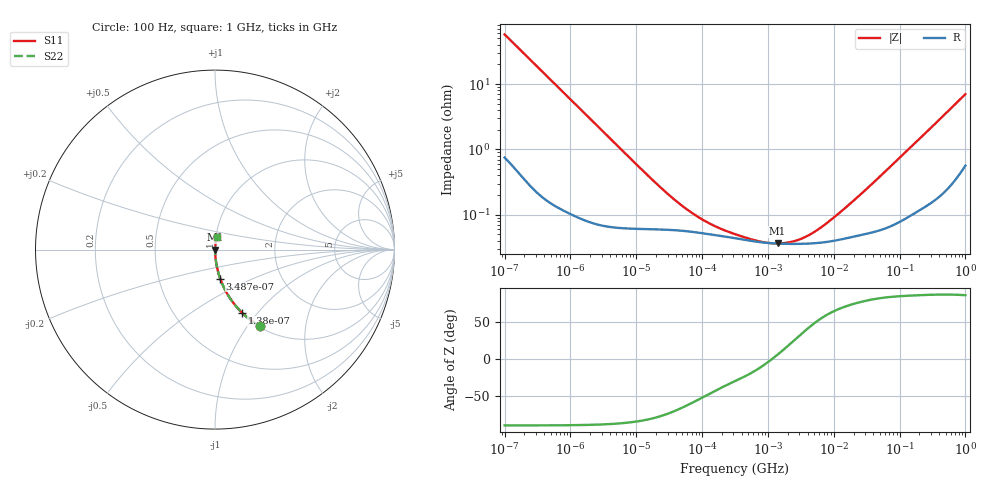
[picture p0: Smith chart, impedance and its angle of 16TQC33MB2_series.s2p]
!  *** S-Parameter ***
!  Copyright (C) Panasonic Industry
!  Conductive Polymer Tantalum Solid Capacitor (POSCAP)
!  Parts No. 16TQC33MB2
!  Connection Mode : Series
!  1  o---||---o  2
!  GND o--------o GND
!  Conditions : Temperature = 20 degC  DC Bias = 0 V
! Frequency Range : 100Hz  -  1GHz  [ 401 Steps ]
# Hz S RI R 50
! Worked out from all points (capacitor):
!   401 points, 100 Hz to 1 GHz, reference 50 ohm
!   read as one part in series: C = 27.6 uF near 108.4 Hz
!   lowest |Z| = 36.3 mohm at 1.404 MHz (marker M1)
!   series resonance near 1.165 MHz, so ESL is about 680 pH
!   S11 on the Smith chart (normalised r, x): 100 Hz: 1.01, -1.15; 138 Hz: 1.01, -0.84; 348.7 Hz: 1.00, -0.33; 1 GHz: 1.01, +0.14
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100  0.2518 -0.4276  0.7482 0.4276  0.7482 0.4276  0.2518 -0.4276
138.0384  0.1522 -0.353  0.8478 0.353  0.8478 0.353  0.1522 -0.353
206.538  0.0756 -0.2585  0.9244 0.2585  0.9244 0.2585  0.0756 -0.2585
348.7386  0.0288 -0.1615  0.9712 0.1615  0.9712 0.1615  0.0288 -0.1615
664.5077  0.00886 -0.0868  0.9911 0.0868  0.9911 0.0868  0.00886 -0.0868
1487.647  0.00239 -0.0392  0.9976 0.0392  0.9976 0.0392  0.00239 -0.0392
4241.31  0.000834 -0.0138  0.9992 0.0138  0.9992 0.0138  0.000834 -0.0138
22130.95  0.000601 -0.00269  0.9994 0.00269  0.9994 0.00269  0.000601 -0.00269
43903.59  0.000575 -0.0014  0.9994 0.0014  0.9994 0.0014  0.000575 -0.0014
83656.56  0.000534 -0.000782  0.9995 0.000782  0.9995 0.000782  0.000534 -0.000782
153108.7  0.000489 -0.000465  0.9995 0.000465  0.9995 0.000465  0.000489 -0.000465
316227.8  0.000437 -0.000251  0.9996 0.000251  0.9996 0.000251  0.000437 -0.000251
737055.2  0.000381 -8.47e-05  0.9996 8.47e-05  0.9996 8.47e-05  0.000381 -8.47e-05
1404430  0.000361 3.6e-05  0.9996 -3.6e-05  0.9996 -3.6e-05  0.000361 3.6e-05
2570396  0.000357 0.000171  0.9996 -0.000171  0.9996 -0.000171  0.000357 0.000171
4704354  0.000364 0.000371  0.9996 -0.000371  0.9996 -0.000371  0.000364 0.000371
7328245  0.00038 0.000594  0.9996 -0.000594  0.9996 -0.000594  0.00038 0.000594
1.34122e7  0.000423 0.00108  0.9996 -0.00108  0.9996 -0.00108  0.000423 0.00108
2.884032e7  0.000504 0.00222  0.9995 -0.00222  0.9995 -0.00222  0.000504 0.00222
6.99842e7  0.000678 0.00523  0.9993 -0.00523  0.9993 -0.00523  0.000678 0.00523
3.368992e8  0.00221 0.0239  0.9978 -0.0239  0.9978 -0.0239  0.00221 0.0239
1e9  0.0104 0.069  0.9896 -0.069  0.9896 -0.069  0.0104 0.069
